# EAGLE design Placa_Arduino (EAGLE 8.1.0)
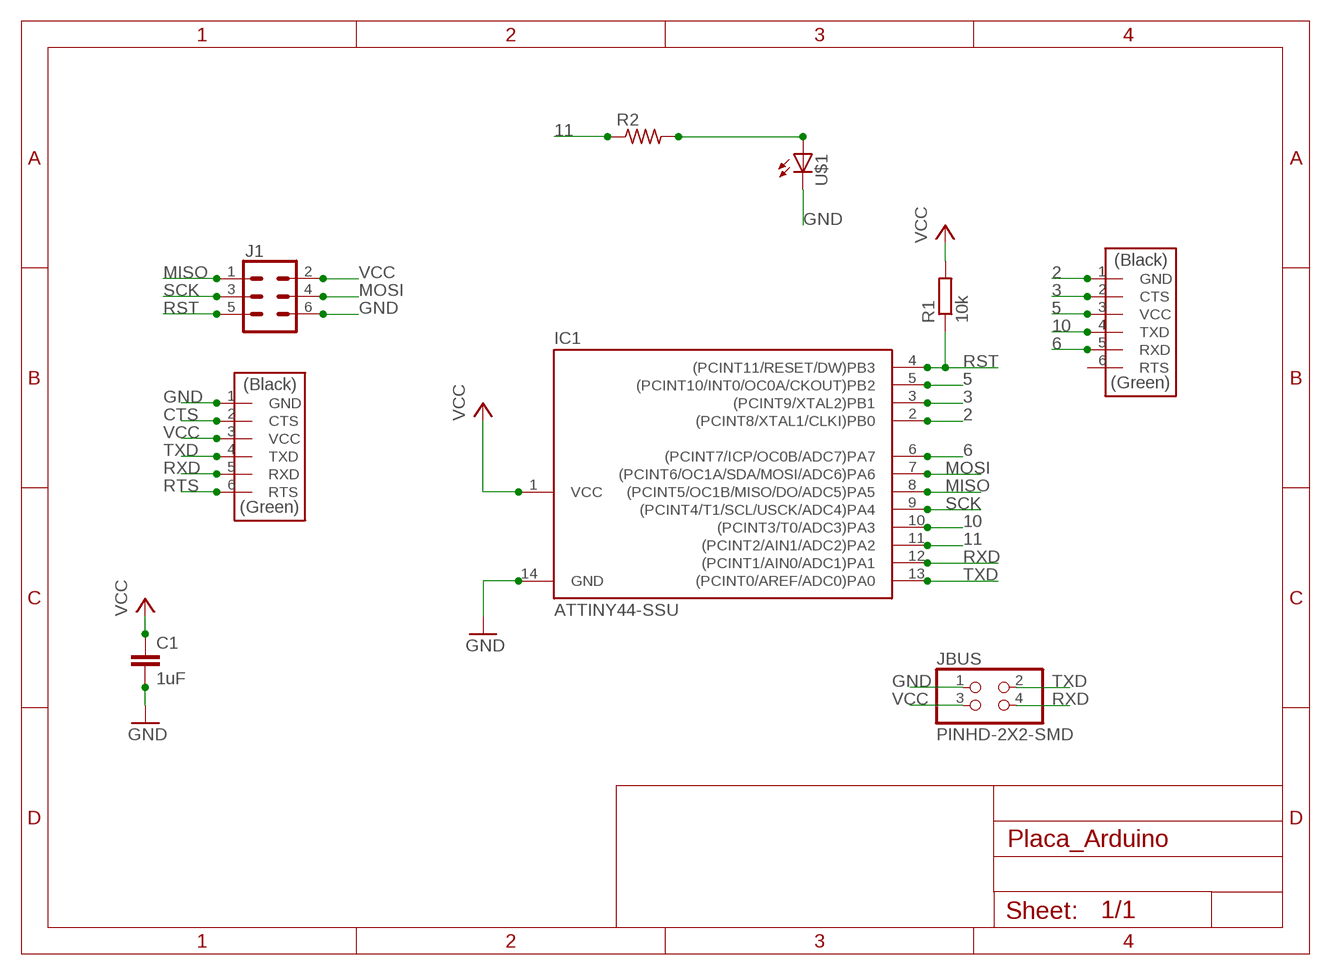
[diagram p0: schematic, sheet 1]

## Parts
C1  1uF  C-EUC1206  [C1206]
IC1  ATTINY44-SSU  [SOIC14]
J1  CONN_03X2SMT  [2X3_SMT_POSTS]
J2  FTDI-SMD-HEADER  [1X06SMD]
J3  FTDI-SMD-HEADER  [1X06SMD]
JBUS  PINHD-2X2-SMD  [2X02SMD]
R1  10k  R-EU_M1206  [M1206]
R2  RESISTOR1206  [1206]
U$1  LED1206  [1206]

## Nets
2: IC1.2((PCINT8/XTAL1/CLKI)PB0) J3.1(GND)
3: IC1.3((PCINT9/XTAL2)PB1) J3.2(CTS)
5: IC1.5((PCINT10/INT0/OC0A/CKOUT)PB2) J3.3(VCC)
6: IC1.6((PCINT7/ICP/OC0B/ADC7)PA7) J3.5(RXD)
10: IC1.10((PCINT3/T0/ADC3)PA3) J3.4(TXD)
11: IC1.11((PCINT2/AIN1/ADC2)PA2) R2.1
CTS: J2.2(CTS)
GND: C1.2 IC1.14(GND) J1.6 J2.1(GND) JBUS.1 U$1.2(C)
MISO: IC1.8((PCINT5/OC1B/MISO/DO/ADC5)PA5) J1.1
MOSI: IC1.7((PCINT6/OC1A/SDA/MOSI/ADC6)PA6) J1.4
N$2: R2.2 U$1.1(A)
RST: IC1.4((PCINT11/RESET/DW)PB3) J1.5 R1.1
RTS: J2.6(RTS)
RXD: IC1.12((PCINT1/AIN0/ADC1)PA1) J2.5(RXD) JBUS.4
SCK: IC1.9((PCINT4/T1/SCL/USCK/ADC4)PA4) J1.3
TXD: IC1.13((PCINT0/AREF/ADC0)PA0) J2.4(TXD) JBUS.2
VCC: C1.1 IC1.1(VCC) J1.2 J2.3(VCC) JBUS.3 R1.2
Unconnected: J3.6(RTS)

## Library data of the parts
C1 = rcl:C-EU: CAPACITOR, European symbol
IC1 = fab:ATTINY44
J1 = SparkFun-Connectors:CONN_03X2: Multi connection point. Often used as Generic Header-pin footprint for 0.1 inch spaced/style header connections You can populate with any combo of single row headers, but if you'd like an exact match, check these: Header - 2x3 (Male, 0.1") (PRT-12807) Header - 2x3 (Female, 0.1") (PRT-13010) 2x3 Pin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; PROD_ID: CONN-11415
J2 J3 = fab:FTDI-SMD-HEADER
JBUS = fab:PINHD-2X2-SMD
R1 = rcl:R-EU_: RESISTOR, European symbol
R2 = FabLab:RESISTOR
U$1 = FabLab:LED

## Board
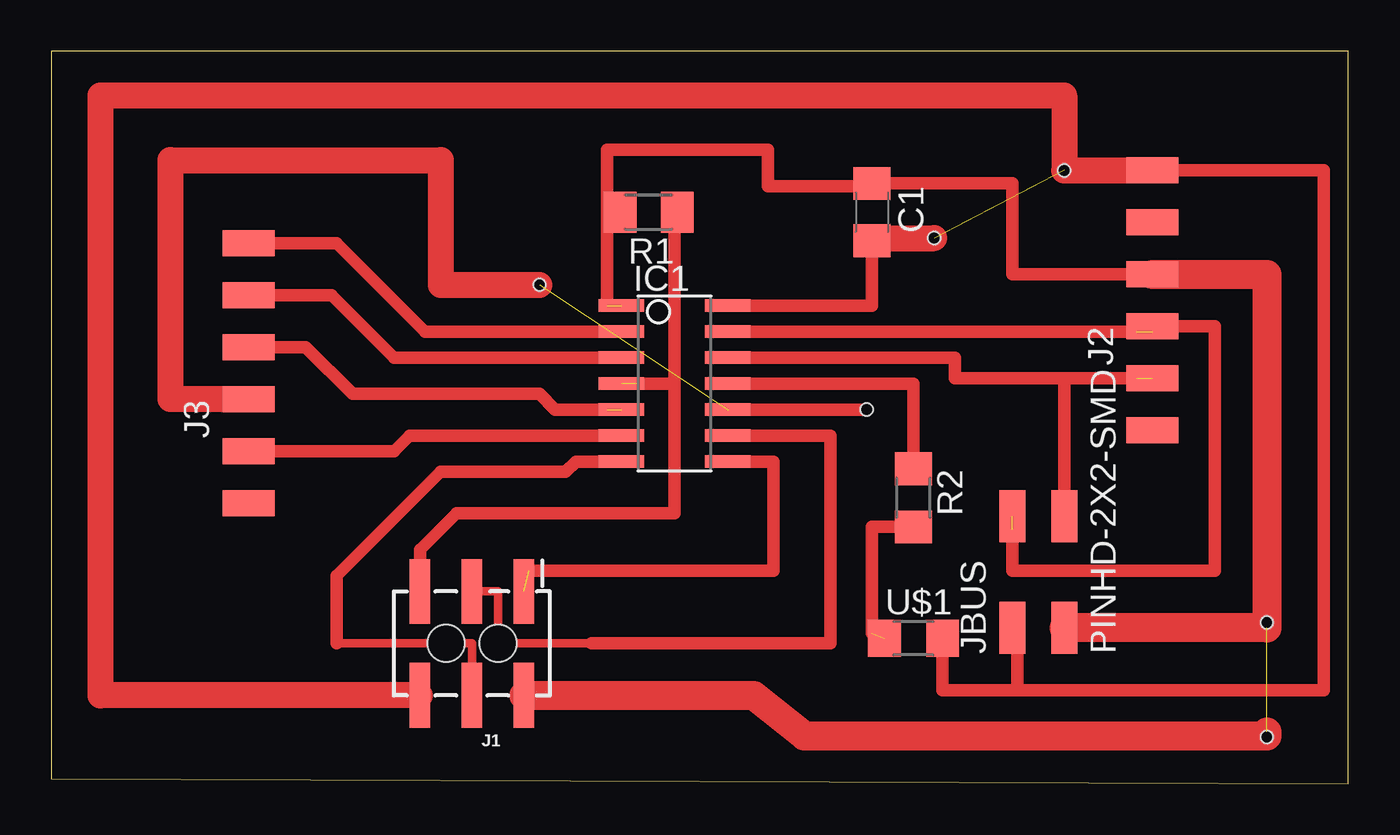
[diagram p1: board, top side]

Size 63.42 x 35.8 mm. Coordinates in mm from the lower left corner, seen from the top.
Outline: 0,0.25 63.42,0 63.42,35.8 0,35.8 0,0.25
Copper layers (1*16): Top 0.035mm / dielectric 1.5mm / Bottom 0.035mm
Design rules "default": minimum track width 10mil, minimum drill 24mil, track to track 8mil, track to pad 8mil, pad to pad 8mil, via to via 8mil, smd to smd 8mil, copper to edge 40mil, drill to drill 8mil, minimum pad ring 10mil, minimum via ring 8mil, stop-mask expansion 4mil, vias tented up to drill 0mil, thermal gap 10mil
Holes 0.6 mm at 23.88,24.38 59.44,2.29 49.53,29.97 43.18,26.67 39.88,18.29 59.44,7.87 59.44,7.87

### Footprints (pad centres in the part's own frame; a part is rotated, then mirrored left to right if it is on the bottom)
C1206 = smd 1.6 x 1.8: 1 -1.4,0; 2 1.4,0
SOIC14 = smd 0.61 x 2.21: 1 -3.81,-2.603; 2 -2.54,-2.603; 3 -1.27,-2.603; 4 0,-2.603; 5 1.27,-2.603; 6 2.54,-2.603; 7 3.81,-2.603; 8 3.81,2.603; 9 2.54,2.603; 10 1.27,2.603; 11 0,2.603; 12 -1.27,2.603; 13 -2.54,2.603; 14 -3.81,2.603
2X3_SMT_POSTS = smd 1 x 3.17: 1 -2.54,-2.54; 2 -2.54,2.54; 3 0,-2.54; 4 0,2.54; 5 2.54,-2.54; 6 2.54,2.54 | hole 1.8: -1.27,0; 1.27,0
1X06SMD = smd 2.54 x 1.27: 1 0,6.35; 2 0,3.81; 3 0,1.27; 4 0,-1.27; 5 0,-3.81; 6 0,-6.35
2X02SMD = smd 2.54 x 1.27: 1 -2.54,1.27; 2 2.92,1.27; 3 -2.54,-1.27; 4 2.92,-1.27
M1206 = smd 1.6 x 2: 1 -1.4,0; 2 1.4,0
1206 = smd 1.6 x 1.803: 1 -1.422,0; 2 1.422,0

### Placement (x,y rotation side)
C1  40.13,27.94 270 top
IC1  30.48,19.56 270 top
J1  20.57,6.86 180 top
J2  53.85,23.62 0 top
J3  9.65,20.07 0 top
JBUS  48.26,10.16 90 top
R1  29.21,27.94 180 top
R2  42.16,13.97 270 top
U$1  42.16,7.11 0 top

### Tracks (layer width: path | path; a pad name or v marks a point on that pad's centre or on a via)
2
  Top 0.61: J3.1 13.97,26.42 18.29,22.1 IC1.2
3
  Top 0.61: J3.2 13.72,23.88 16.76,20.83 IC1.3
5  (1 unrouted)
  Top 0.61: J3.3 12.45,21.34 14.73,19.05 23.88,19.05 24.64,18.29 27.18,18.29
6
  Top 0.61: J3.5 16.76,16.26 17.53,17.02 IC1.6
10  (1 unrouted)
  Top 0.61: IC1.10 39.62,18.29
  Top 1.27: J3.4 5.84,18.8 5.84,30.48 19.05,30.48 19.05,24.38 23.88,24.38
11
  Top 0.61: IC1.11 42.16,19.56 R2.1
GND  (1 unrouted)
  Top 0.406: C1.2 40.26,26.67
  Top 0.61: IC1.14 40.13,23.37 C1.2 | J2.1 62.23,29.97 62.23,4.57 47.24,4.57 | U$1.2 43.59,4.57 47.24,4.57 | JBUS.1 47.24,7.62 47.24,4.57
  Top 1.27: 40.26,26.67 43.18,26.67 | J1.6 2.41,4.32 2.41,33.64 49.53,33.64 49.53,29.97 J2.1
MISO  (1 unrouted)
  Top 0.61: IC1.8 35.31,15.75 35.31,10.41 23.37,10.41
MOSI
  Top 0.406: 13.97,6.86 20.57,6.86 J1.4
  Top 0.61: IC1.7 25.65,15.75 25.15,15.24 19.05,15.24 13.97,10.16 13.97,6.86
N$2  (1 unrouted)
  Top 0.61: R2.2 40.13,12.55 40.13,7.37
RST  (1 unrouted)
  Top 0.61: R1.1 30.48,27.94 30.48,19.56 | 30.48,19.56 28.7,19.56 | J1.5 18.03,11.43 19.81,13.21 30.48,13.21 30.48,19.56
RXD  (1 unrouted)
  Top 0.61: IC1.12 44.2,20.83 44.2,19.81 49.53,19.81 | 49.53,19.81 53.09,19.81 | JBUS.4 49.53,19.81
SCK
  Top 0.406: 26.42,6.86 21.84,6.86 21.84,9.4 J1.3
  Top 0.61: IC1.9 38.1,17.02 38.1,6.86 26.42,6.86
TXD  (2 unrouted)
  Top 0.406: 53.85,22.1 J2.4
  Top 0.61: IC1.13 53.09,22.1 | J2.4 56.9,22.35 56.9,10.41 46.99,10.41 46.99,12.45
VCC  (2 unrouted)
  Top 0.406: IC1.1 27.94,23.37
  Top 0.61: 27.18,27.94 27.18,23.37 | R1.2 27.18,27.94 | 27.18,27.94 27.18,30.99 35.05,30.99 35.05,29.21 40.13,29.21 C1.1 46.99,29.34 46.99,24.89 J2.3
  Top 1.422: J2.3 59.44,24.89 59.44,7.62 JBUS.3 | J1.2 34.35,4.32 36.83,2.34 59.44,2.34 59.44,2.54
